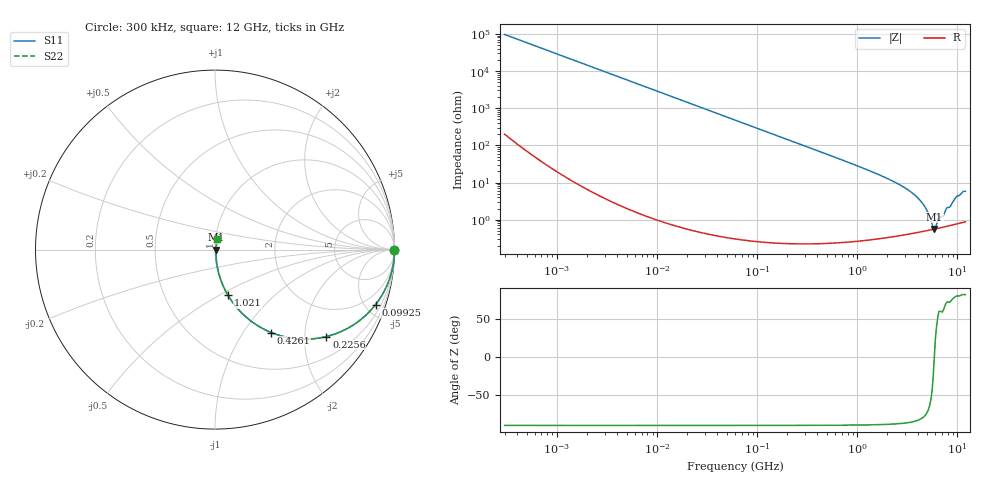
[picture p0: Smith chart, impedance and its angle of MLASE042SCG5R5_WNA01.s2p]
! MLASE042SCG5R5_WNA01  S-PARAMETER MODEL  ( General Type )
! Model Generated by TAIYO YUDEN Corporation (http://www.ty-top.com)
! Version 1.0
! TAIYO YUDEN Control No. 130801
! Copyright(c) 2013 TAIYO YUDEN CO.,LTD. All Rights Reserved.
! Product Description (link to TY-COMPAS)
! https://ds.yuden.co.jp/TYCOMPAS/or/detail?pn=MLASE042SCG5R5BWNA01&u=M
! Products Name : Multilayer Ceramic Capacitors
! Characteristics :
!  Capacitance : 5.5 pF , Rated Voltage : 16V , TCC : CG / C0G
!  Case Size : 0.4 x 0.2 / 0.016 x 0.008 [mm/inch] , Thickness : 0.2 / 0.008 [mm/inch]
!  (Conditions: Temperature = 25 degC , DC Bias Current/Voltage = 0A / 0V)
! External Node Assignments :
!  1  o---| |---o  2
! GND o---------o GND
! Frequency Range : 0.3MHz  -  12000MHz  [ 401 STEP ]
# MHz S RI R 50
! Freq[MHz].  S11 Real  S11 Imag  S21 Real  S21 Imag  S12 Real  S12 Imag  S22 Real  S22 Imag
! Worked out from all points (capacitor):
!   401 points, 300 kHz to 12 GHz, reference 50 ohm
!   read as one part in series: C = 5.5 pF near 316.3 kHz
!   lowest |Z| = 559 mohm at 5.869 GHz (marker M1)
!   series resonance near 5.884 GHz, so ESL is about 130 pH
!   S11 on the Smith chart (normalised r, x): 300 kHz: open; 99.25 MHz: 1.01, -5.83; 225.6 MHz: 1.00, -2.56; 426.1 MHz: 1.00, -1.35; 1.021 GHz: 1.01, -0.55; 12 GHz: 1.02, +0.12
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0.3  1 -0.00104  3.23e-06 0.00104  3.23e-06 0.00104  1 -0.00104
1.769972  1 -0.00612  4.04e-05 0.00612  4.04e-05 0.00612  1 -0.00612
10.44266  0.9987 -0.0361  0.00131 0.0361  0.00131 0.0361  0.9987 -0.0361
27.82928  0.9908 -0.0953  0.00921 0.0953  0.00921 0.0953  0.9908 -0.0953
60  0.9586 -0.1989  0.0414 0.1989  0.0414 0.1989  0.9586 -0.1989
99.25425  0.8944 -0.3069  0.1056 0.3069  0.1056 0.3069  0.8944 -0.3069
147.6816  0.7927 -0.4048  0.2073 0.4048  0.2073 0.4048  0.7927 -0.4048
225.6362  0.6208 -0.4843  0.3792 0.4843  0.3792 0.4843  0.6208 -0.4843
353.9943  0.3989 -0.4883  0.6011 0.4883  0.6011 0.4883  0.3989 -0.4883
426.1204  0.3137 -0.4623  0.6863 0.4623  0.6863 0.4623  0.3137 -0.4623
651.0506  0.1628 -0.3665  0.8372 0.3665  0.8372 0.3665  0.1628 -0.3665
1021.415  0.0722 -0.2541  0.9278 0.2541  0.9278 0.2541  0.0722 -0.2541
2088.533  0.0176 -0.1185  0.9824 0.1185  0.9824 0.1185  0.0176 -0.1185
3107.553  0.00841 -0.0663  0.9916 0.0663  0.9916 0.0663  0.00841 -0.0663
4050.141  0.00593 -0.0372  0.9941 0.0372  0.9941 0.0372  0.00593 -0.0372
4747.894  0.00538 -0.0211  0.9946 0.0211  0.9946 0.0211  0.00538 -0.0211
5140.631  0.00533 -0.0132  0.9947 0.0132  0.9947 0.0132  0.00533 -0.0132
5565.855  0.00541 -0.00545  0.9946 0.00545  0.9946 0.00545  0.00541 -0.00545
5868.704  0.00555 -0.000267  0.9944 0.000267  0.9944 0.000267  0.00555 -0.000267
6524.734  0.006 0.00989  0.994 -0.00989  0.994 -0.00989  0.006 0.00989
9454.42  0.00871 0.0358  0.9913 -0.0358  0.9913 -0.0358  0.00871 0.0358
12000  0.0119 0.0564  0.9881 -0.0564  0.9881 -0.0564  0.0119 0.0564
